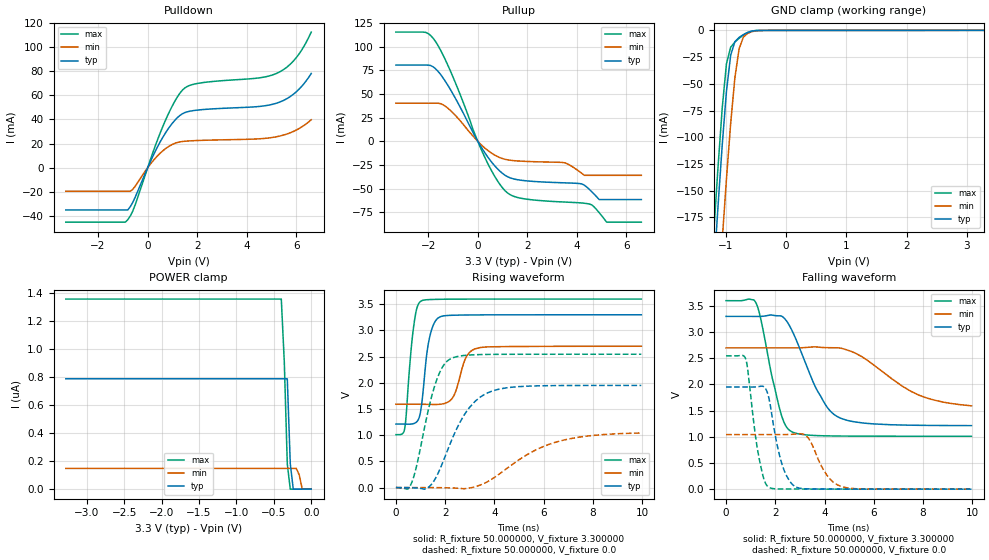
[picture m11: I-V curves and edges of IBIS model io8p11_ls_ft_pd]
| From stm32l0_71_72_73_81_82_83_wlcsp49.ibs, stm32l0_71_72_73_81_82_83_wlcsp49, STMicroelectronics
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|   Model io8p11_ls_ft_pd
[Model]  io8p11_ls_ft_pd
Model_type I/O
Polarity   Non-Inverting
Enable   Active-Low
Vinl =   0.990000V
Vinh =   2.310000V
Vmeas =  1.650000V
Cref =   50.000000pF
Rref =   100.000000M
Vref =   0.0V
C_comp   4.606100pF   4.563500pF   4.706200pF
[Temperature Range]   25.000000   0.125000k   -40.000000
[Pullup Reference]   3.300000V   2.700000V   3.600000V
[Pulldown Reference]   0.0V   0.0V   0.0V
[POWER Clamp Reference]   3.300000V   2.700000V   3.600000V
[GND Clamp Reference]   0.0V   0.0V   0.0V
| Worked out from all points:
|   slope of the pulldown table from 0 to 0.495 V, typ, clamps not added: 23.6 ohm
|   slope of the pullup table from 0 to 0.495 V, typ, clamps not added: 24.9 ohm
|   GND clamp passes 1 mA (typ) near -0.59 V on its own axis
|   rising waveform, R_fixture 50.000000, V_fixture 3.300000: 20-80 % time 320ps typ, 430ps min, 283ps max; typ from 1.21 V to 3.3 V
|   rising waveform, R_fixture 50.000000, V_fixture 0.0: 20-80 % time 1.23ns typ, 2.23ns min, 756ps max; typ from 0 V to 1.95 V
|   falling waveform, R_fixture 50.000000, V_fixture 3.300000: 20-80 % time 1.19ns typ, 2.07ns min, 695ps max; typ from 3.3 V to 1.21 V
|   falling waveform, R_fixture 50.000000, V_fixture 0.0: 20-80 % time 522ps typ, 686ps min, 437ps max; typ from 1.95 V to 0 V
[Pulldown]
|Voltage   I(typ)   I(min)   I(max)
-3.3V     -34.78mA   -19.34mA   -44.89mA
-900mV    -34.78mA   -19.34mA   -44.89mA
-800mV    -34.78mA   -19.34mA   -42.84mA
-600mV    -28.56mA   -17.8mA    -35.74mA
100mV     4.638mA    2.744mA    6.076mA
600mV     24.8mA     13.84mA    33.52mA
1V        36.92mA    19.39mA    51.35mA
1.4V      44.67mA    21.76mA    64.17mA
2V        47.7mA     22.58mA    69.7mA
5.2V      53.44mA    25.71mA    78.04mA
6V        62.89mA    31.28mA    91.14mA
6.6V      77.95mA    39.75mA    112.2mA
[Pullup]
|Voltage   I(typ)   I(min)   I(max)
-3.3V     80.5mA     40.22mA    115.4mA
-2.1V     80.5mA     40.22mA    115.1mA
-1.7V     76.61mA    40.22mA    105.3mA
-1.1V     54.57mA    32.56mA    74.14mA
300mV     -12.7mA    -7.45mA    -17.83mA
800mV     -29.19mA   -16.17mA   -41.96mA
1.2V      -37.42mA   -19.62mA   -54.57mA
3.5V      -43.95mA   -22.7mA    -64.24mA
4.5V      -50.83mA   -35.99mA   -66.3mA
4.9V      -61.63mA   -35.99mA   -75.5mA
5.2V      -61.63mA   -35.99mA   -85.54mA
6.6V      -61.63mA   -35.99mA   -85.54mA
[GND_clamp]
|Voltage   I(typ)   I(min)   I(max)
-3.3V     -2.275A    -2.356A    -2.249A
-1.2V     -226mA     -318.7mA   -189.2mA
-1.13V    -164.9mA   -256.6mA   -128.3mA
-1.06V    -107.5mA   -196.5mA   -72.79mA
-990mV    -57.33mA   -139.4mA   -31.4mA
-920mV    -23.23mA   -87.33mA   -15.73mA
-850mV    -10.59mA   -44.46mA   -10.94mA
-780mV    -6.551mA   -17.26mA   -7.364mA
-710mV    -3.945mA   -6.365mA   -4.316mA
-640mV    -1.966mA   -2.806mA   -1.983mA
-360mV    -10.16uA   -28.12uA   -6.105uA
3.28V     73.92uA    88.6uA     51.45uA
[POWER_clamp]
|Voltage   I(typ)   I(min)   I(max)
-3.28V    786.7nA    148nA      1.355uA
-400mV    786.7nA    148nA      1.355uA
-360mV    786.7nA    148nA      908.2nA
-320mV    786.7nA    148nA      180.5nA
-280mV    182.6nA    148nA      0A
-240mV    0A         148nA      0A
-200mV    0A         148nA      0A
-160mV    0A         101.6nA    0A
-120mV    0A         0A         0A
0V        0A         0A         0A
[Ramp]
| variable   typ   min   max
dV/dt_r  1.16985/1.22368n   0.60665/2.14806n   1.52706/0.75481n
dV/dt_f  1.24914/1.19115n   0.57846/1.85895n   1.55256/0.69347n
R_load = 50.000000
[Rising Waveform]
R_fixture= 50.000000
V_fixture= 3.300000
V_fixture_min= 2.700000
V_fixture_max= 3.600000
|time   V(typ)   V(min)   V(max)
0s        1.213V     1.591V     1.01V
360.4ps   1.212V     1.591V     1.135V
720.7ps   1.222V     1.591V     3.074V
1.041ns   1.576V     1.59V      3.565V
1.361ns   2.853V     1.588V     3.589V
1.802ns   3.26V      1.591V     3.594V
2.342ns   3.29V      1.744V     3.597V
2.843ns   3.294V     2.481V     3.598V
3.223ns   3.296V     2.649V     3.598V
9.97ns    3.298V     2.698V     3.598V
[Rising Waveform]
R_fixture= 50.000000
V_fixture= 0.0
V_fixture_min= 0.0
V_fixture_max= 0.0
|time   V(typ)   V(min)   V(max)
0s        415.7uV    51.65uV    -108.3uV
620.6ps   -2.248mV   116.3uV    72.41mV
1.221ns   -21.76mV   300.6uV    1.278V
1.582ns   156.7mV    -214.1uV   1.952V
1.882ns   456.8mV    -2.23mV    2.293V
2.202ns   836.7mV    -6.106mV   2.453V
2.983ns   1.526V     -9.148mV   2.53V
3.924ns   1.844V     169.9mV    2.542V
6.406ns   1.946V     854.2mV    2.545V
9.97ns    1.95V      1.042V     2.545V
[Falling Waveform]
R_fixture= 50.000000
V_fixture= 3.300000
V_fixture_min= 2.700000
V_fixture_max= 3.600000
|time   V(typ)   V(min)   V(max)
0s        3.298V     2.698V     3.598V
1.221ns   3.297V     2.698V     3.55V
1.401ns   3.298V     2.698V     3.267V
2.202ns   3.309V     2.698V     1.49V
2.663ns   3.043V     2.697V     1.099V
3.684ns   1.901V     2.715V     1.023V
4.545ns   1.379V     2.699V     1.015V
5.506ns   1.267V     2.533V     1.012V
7.848ns   1.219V     1.792V     1.01V
9.97ns    1.213V     1.591V     1.01V
[Falling Waveform]
R_fixture= 50.000000
V_fixture= 0.0
V_fixture_min= 0.0
V_fixture_max= 0.0
|time   V(typ)   V(min)   V(max)
0s        1.95V      1.042V     2.545V
800.8ps   1.95V      1.042V     2.48V
1.321ns   1.958V     1.042V     644.3mV
1.762ns   1.69V      1.042V     30.14mV
2.282ns   462.1mV    1.042V     3.623mV
2.863ns   36.09mV    1.055V     2.287mV
3.323ns   5.325mV    984.9mV    1.518mV
4.104ns   2.698mV    263.5mV    711.1uV
4.665ns   2.038mV    55.12mV    392.6uV
9.97ns    415.7uV    51.65uV    -108.3uV
